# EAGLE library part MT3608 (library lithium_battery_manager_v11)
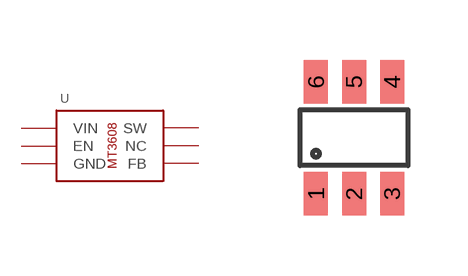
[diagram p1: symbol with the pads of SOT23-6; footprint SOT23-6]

Designator prefix -

## MT3608  [SOT23-6]
1  SW
2  GND
3  FB
4  EN
5  VIN
6  NC

## Footprint SOT23-6 (pad centres in mm)
SOT23-6
smd 0.6 x 1.1: 1 0,0; 2 0.95,0; 3 1.9,0; 4 1.9,2.8; 5 0.95,2.8; 6 0,2.8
